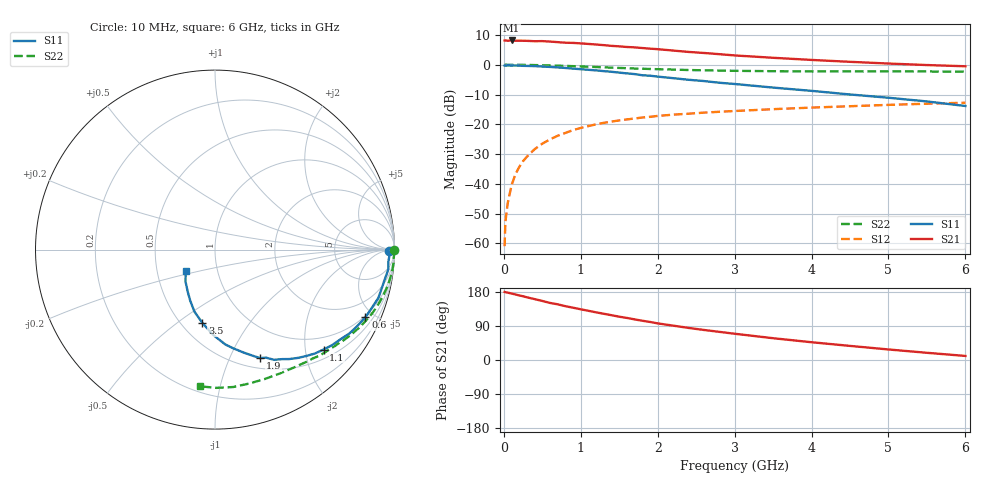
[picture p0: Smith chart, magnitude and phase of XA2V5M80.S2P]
! SIEMENS Discrete & RF Semiconductors
! BFY180
! Si NPN RF Bipolar Junction Transistor in MICRO-X
! VCE = 2.5 V  IC = 0.8 mA
! Common Emitter S-Parameters:  May  1997
# GHz  S  MA  R  50
!  f  S11  S21  S12  S22
! GHz  MAG  ANG  MAG  ANG  MAG  ANG  MAG  ANG
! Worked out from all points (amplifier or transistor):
!   36 points, 10 MHz to 6 GHz, reference 50 ohm
!   highest |S21| = 8.2 dB at 100 MHz (marker M1)
!   |S21| within 3 dB of that: start of sweep to 2.032 GHz
!   unconditionally stable (mu >= 1): 4.143 GHz to end of sweep
!   at 250 MHz: K = 0.06, MSG = 20.2 dB, |S12| = -32.4 dB
!   at 1.4 GHz: K = 0.47, MSG = 12.7 dB, |S12| = -19.1 dB
!   at 6 GHz: K = 1.06, MAG = 4.6 dB, |S12| = -12.8 dB
!   S11 on the Smith chart (normalised r, x): 10 MHz: 64, -15; 600 MHz: 0.92, -4.48; 1.1 GHz: 0.70, -2.39; 1.9 GHz: 0.62, -1.31; 3.5 GHz: 0.63, -0.62; 6 GHz: 0.70, -0.18
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0.01  0.971 -0.4  2.549 179.6  0.0009 94.2  0.9984 -0.2
0.02  0.9606 -1.0  2.555 178.9  0.0023 83.4  0.9999 -0.5
0.05  0.9722 -2.0  2.527 177.8  0.0047 86.3  0.9983 -1.3
0.1  0.9681 -4.2  2.556 175.4  0.0095 86.5  0.997 -2.6
0.15  0.9718 -6.5  2.529 173.0  0.0144 85.1  0.9988 -3.9
0.25  0.9585 -10.6  2.525 168.2  0.0241 83.0  0.9953 -6.5
0.4  0.9491 -16.5  2.483 160.7  0.0382 78.4  0.9873 -10.1
0.5  0.9316 -20.5  2.491 155.8  0.0473 75.5  0.9804 -12.6
0.6  0.9192 -24.2  2.45 150.6  0.0558 72.7  0.9727 -14.9
0.9  0.8603 -35.4  2.326 138.0  0.0799 64.1  0.9462 -21.8
1.1  0.8223 -42.6  2.233 129.8  0.0934 59.3  0.925 -26.0
1.5  0.7373 -55.8  2.037 114.3  0.1162 50.7  0.884 -33.8
1.7  0.6969 -61.8  1.958 107.2  0.1252 47.3  0.8635 -37.3
1.9  0.6546 -67.4  1.863 100.4  0.1334 43.9  0.8485 -40.5
2.2  0.5952 -74.5  1.73 90.7  0.1452 39.4  0.8301 -45.3
2.4  0.5594 -79.5  1.641 84.7  0.1506 37.0  0.8151 -48.1
2.8  0.4989 -87.8  1.505 74.3  0.1623 32.7  0.7973 -53.5
3.5  0.4135 -99.9  1.308 57.5  0.1795 26.1  0.7788 -62.6
4  0.3644 -108.3  1.204 46.9  0.1908 21.7  0.7724 -69.0
4.5  0.3168 -115.8  1.119 37.2  0.2011 17.8  0.7701 -75.7
5.5  0.242 -132.8  0.988 19.0  0.2217 9.7  0.7704 -89.5
6  0.203 -143.7  0.942 10.7  0.2303 5.5  0.7662 -96.4
